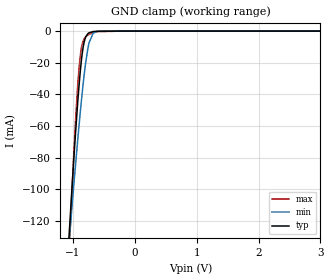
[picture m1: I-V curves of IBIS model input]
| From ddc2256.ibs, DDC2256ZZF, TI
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|   input Model
[Model]   input
Model_type   Input
Vinl = 0.54
Vinh = 1.26
|   typ   min   max
|   (nom PVT)   (fast PVT)   (slow PVT)
C_comp   9.690e-13   9.585e-13   9.818e-13
| Where nom  PVT is Nominal Process, 1.8V, 27C
|   Fast PVT is Strong Process,  1.9V, 0C
|   Slow PVT is Weak Process,   1.7V, 85C
[Voltage Range]   1.8   1.7   1.9
|Junction Temperature
[Temperature Range]   27   85   0
[Power Clamp Reference]   1.8   1.7   1.9
[GND Clamp Reference]   0   0   0
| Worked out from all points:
|   GND clamp passes 1 mA (typ) near -0.73 V on its own axis
[GND Clamp]
|   Voltage   I(typ)   I(min)   I(max)
-1.8V     -657.3mA   -511.7mA   -867.5mA
-1.057V   -126.7mA   -131.4mA   -137.6mA
-1.015V   -100.1mA   -111.8mA   -102.2mA
-960.2mV  -66.58mA   -86.24mA   -59.17mA
-924.5mV  -46.74mA   -70.31mA   -35.87mA
-889.9mV  -29.82mA   -55.52mA   -19.06mA
-858.2mV  -17.32mA   -42.74mA   -9.916mA
-820.8mV  -7.566mA   -29mA      -5.16mA
-739.2mV  -1.092mA   -7.547mA   -2.13mA
-671.2mV  -303.7uA   -1.268mA   -1.003mA
-603mV    -81.56uA   -165.3uA   -364.5uA
3.6V      0A         0A         0A
[POWER Clamp]
|   Voltage   I(typ)   I(min)   I(max)
-1.8V     0A         0A         0A
0V        0A         0A         0A
3.6V      0A         0A         0A
